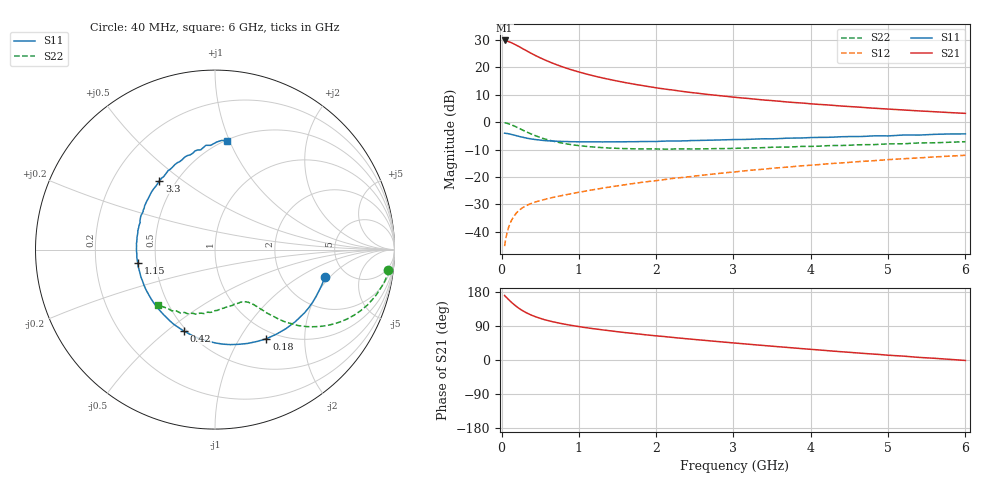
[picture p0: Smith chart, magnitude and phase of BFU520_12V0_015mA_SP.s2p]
! Filename:  P:\Prog\Test\Noise\ATS_data\Testdata_Net\03 Spar\BFU520_APG2013_37_A05_12p0V_015mA_SP_CM01_D.s2p
! Date/Time: Fri 26/Apr/2013 13:00:11
! BFU520_APG2013_37_A05_12p0V_1to20mA_SP_CM01_Bias7_R.s2p
! MDIF S-parameter v. bias file
! BFU520_APG2013_37_A05_12p0V_1to20mA_SP_CM01
! Date/time Tue Apr 23 18:22:57 2013
! VAR V_out= 12.0010
! VAR I_out= 14.9900
! VAR V_in= 0.8015
! VAR I_in= 0.1535
! Device data file deembeded for feedlines and parallel
! Original file: \03 Spar\BFU520_APG2013_37_A05_12p0V_015mA_SP_CM01_R.s2p
! Feed-files: PR047V01_250413_Feed1.s2p, PR047V01_250413_Feed2.s2p
! Parallel-file: PR047V01_250413_Par.s2p
# MHz S MA R 50
!  Freq-MHz  S11-mag  S11-arg  S21-mag  S21-arg  S12-mag  S12-arg  S22-mag  S22-arg
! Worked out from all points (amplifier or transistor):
!   98 points, 40 MHz to 6 GHz, reference 50 ohm
!   highest |S21| = 29.8 dB at 40 MHz (marker M1)
!   |S21| within 3 dB of that: start of sweep to 274.4 MHz
!   unconditionally stable (mu >= 1): 1.627 GHz to 3.769 GHz
!   at 300 MHz: K = 0.38, MSG = 28.6 dB, |S12| = -30.7 dB
!   at 1.6 GHz: K = 1.00, MSG = 18.6 dB, |S12| = -22.8 dB
!   at 6 GHz: K = 0.86, MSG = 7.6 dB, |S12| = -12.1 dB
!   S11 on the Smith chart (normalised r, x): 40 MHz: 3.44, -1.77; 180 MHz: 0.89, -1.31; 420 MHz: 0.48, -0.58; 1.15 GHz: 0.39, -0.07; 3.3 GHz: 0.41, +0.41; 6 GHz: 0.51, +0.98
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40  0.6304 -14.2  30.79 170.3  0.005498 80.9  0.973 -6.6
50  0.6274 -17.9  30.79 167.5  0.006814 79.9  0.9697 -8.6
120  0.6014 -41.9  28.32 153.8  0.01526 71.7  0.9036 -20.0
140  0.5918 -48.2  27.47 150.1  0.01732 69.4  0.8795 -22.8
180  0.5732 -60.1  25.75 143.4  0.02107 65.3  0.8303 -27.8
240  0.5439 -75.9  23.21 134.3  0.02556 60.6  0.7557 -34.0
300  0.5206 -89.4  20.85 127.0  0.0291 57.3  0.6883 -38.6
360  0.5016 -101.0  18.72 120.9  0.03196 55.0  0.6303 -42.2
420  0.4863 -110.7  16.89 115.7  0.03439 53.6  0.58 -44.8
480  0.4749 -119.2  15.33 111.3  0.03656 52.6  0.5389 -46.9
550  0.4624 -128.0  13.81 106.8  0.03874 52.2  0.4978 -48.6
650  0.4531 -137.9  12.04 101.6  0.04202 52.0  0.4567 -50.7
800  0.4447 -149.8  10.05 95.2  0.04661 52.6  0.4115 -52.8
1050  0.4376 -165.2  7.85 86.6  0.05431 54.0  0.3673 -55.7
1150  0.4368 -170.0  7.207 83.7  0.05749 54.5  0.3558 -56.6
1600  0.4387 171.9  5.257 72.3  0.07244 56.0  0.3298 -62.3
2050  0.4479 159.1  4.123 62.8  0.08768 56.4  0.3232 -69.1
3100  0.483 133.1  2.768 43.3  0.1276 54.1  0.336 -86.4
3300  0.4931 128.9  2.607 39.8  0.1357 53.2  0.34 -89.7
4100  0.5274 113.3  2.107 26.6  0.1684 48.8  0.3644 -103.6
5200  0.5832 95.0  1.666 10.2  0.2153 41.2  0.4038 -122.4
6000  0.6108 83.7  1.445 -1.2  0.249 34.6  0.4403 -135.7
